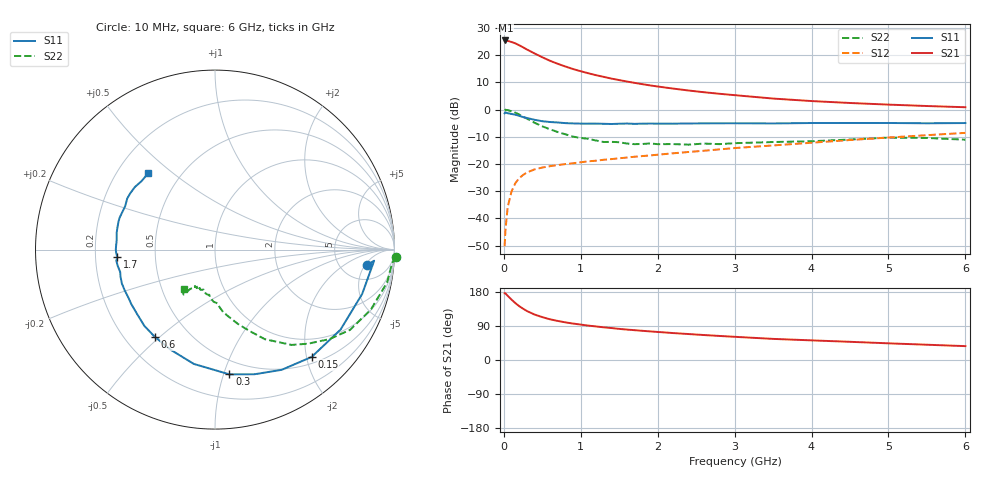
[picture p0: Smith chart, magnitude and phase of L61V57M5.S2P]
!  INFINEON TECHNOLOGIES Small Signal Semiconductors
! BFR380L3 , Si-NPN RF-Transistor in TSLP-3-1
!  Vce=1.5 V,  Ic=7.5 mA
! Common Emitter S-Parameters:  07. March 2005
#  GHz  S  MA  R  50
! f  S11  S21  S12  S22
! GHz  Mag  Ang  Mag  Ang  Mag  Ang  Mag  Ang
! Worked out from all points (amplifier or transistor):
!   36 points, 10 MHz to 6 GHz, reference 50 ohm
!   highest |S21| = 25.4 dB at 20 MHz (marker M1)
!   |S21| within 3 dB of that: start of sweep to 280.3 MHz
!   unconditionally stable (mu >= 1): 2.257 GHz to 4.844 GHz
!   at 250 MHz: K = 0.22, MSG = 23.4 dB, |S12| = -24.0 dB
!   at 1.4 GHz: K = 0.84, MSG = 14.8 dB, |S12| = -18.2 dB
!   at 6 GHz: K = 0.97, MSG = 4.7 dB, |S12| = -8.6 dB
!   S11 on the Smith chart (normalised r, x): 10 MHz: 9, -6; 150 MHz: 0.62, -2.10; 300 MHz: 0.38, -1.05; 600 MHz: 0.32, -0.48; 1.7 GHz: 0.29, -0.04; 6 GHz: 0.33, +0.41
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0.01  0.8526 -5.7  18.52 176.1  0.0031 89.3  1.008 -2.2
0.02  0.8888 -4.0  18.57 176.0  0.0059 89.0  0.9889 -4.5
0.05  0.8563 -16.8  18.24 169.3  0.0162 83.0  0.9762 -10.8
0.1  0.8294 -32.5  17.38 159.4  0.0313 74.6  0.9307 -21.0
0.15  0.8048 -48.0  16.41 150.0  0.0446 66.7  0.8755 -30.7
0.2  0.7659 -61.0  15.13 142.0  0.0551 61.9  0.8099 -38.0
0.25  0.7285 -72.4  13.9 135.4  0.0629 56.3  0.7374 -45.3
0.3  0.6998 -83.4  12.68 129.2  0.0699 53.1  0.6815 -51.2
0.4  0.6478 -100.5  10.71 119.9  0.0797 48.0  0.5714 -60.9
0.5  0.6105 -113.7  9.127 113.1  0.0861 45.3  0.4915 -67.1
0.6  0.5905 -124.6  7.865 107.4  0.0913 43.5  0.434 -72.8
0.7  0.5793 -132.8  6.926 103.1  0.0955 43.5  0.387 -77.8
0.8  0.5632 -140.4  6.171 99.3  0.0998 42.9  0.3513 -82.6
1.1  0.552 -155.9  4.63 90.7  0.1122 44.8  0.2899 -91.7
1.4  0.5428 -166.7  3.7 84.3  0.1232 46.7  0.2553 -98.3
1.7  0.546 -175.5  3.089 78.7  0.1361 49.2  0.2315 -106.1
2.2  0.5505 174.0  2.429 71.1  0.1573 52.2  0.2322 -111.3
2.8  0.5598 163.7  1.95 63.5  0.1853 55.4  0.2317 -118.9
3.5  0.556 154.1  1.592 55.7  0.2193 56.5  0.2533 -121.3
4.5  0.5669 146.4  1.32 48.0  0.2756 58.2  0.2813 -123.7
5.5  0.5596 137.0  1.161 40.3  0.3386 56.9  0.3008 -126.2
6  0.5652 131.3  1.103 36.6  0.373 55.5  0.2794 -128.8
